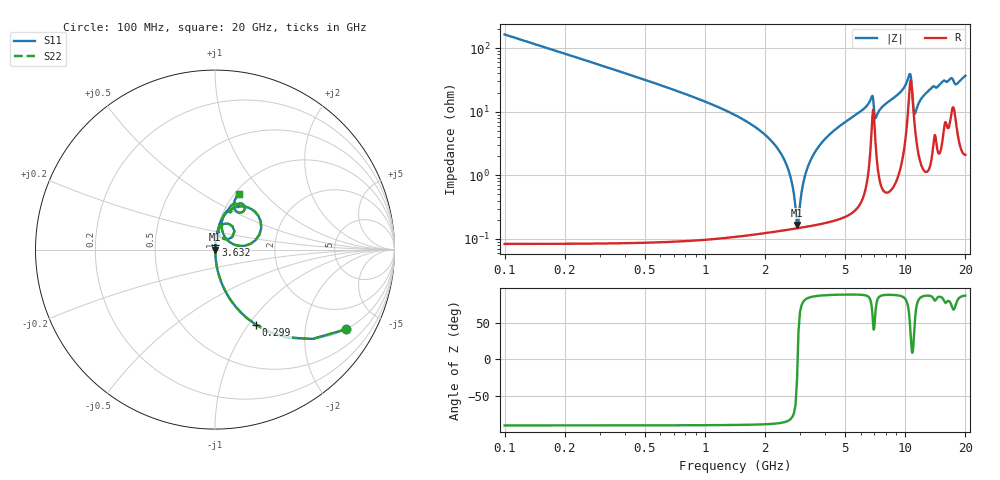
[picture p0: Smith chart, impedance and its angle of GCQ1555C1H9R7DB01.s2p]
!Murata Part Number: GCQ1555C1H9R7DB01
!These Parameters are Measured in Series Mode Connection
!Data Generated on Mar 13, 2026
!  o--ll--o
!Port1  Port2
!  o------o
!Operation Temp=25[degC], DC Bias Voltage=0[V]
!Freq. Start=100[MHz] Stop=20[GHz] 401[Steps]
# Hz S RI R 50
!Freq.(Hz) S11(Real) S11(Imag) S21(Real) S21(Imag) S12(Real) S12(Imag) S22(Real) S22(Imag)
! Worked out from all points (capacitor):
!   401 points, 100 MHz to 20 GHz, reference 50 ohm
!   read as one part in series: C = 9.7 pF near 199.5 MHz
!   lowest |Z| = 165 mohm at 2.886 GHz (marker M1)
!   series resonance near 2.905 GHz, so ESL is about 310 pH
!   S11 on the Smith chart (normalised r, x): 100 MHz: 1.00, -3.28; 299 MHz: 1.00, -1.09; 3.632 GHz: 1.00, +0.05; 20 GHz: 1.04, +0.74
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1e8  0.7286 -0.4444  0.2714 0.4444  0.2714 0.4444  0.7286 -0.4444
2.99e8  0.228 -0.4188  0.772 0.4188  0.772 0.4188  0.228 -0.4188
7.4675e8  0.0412 -0.1966  0.9588 0.1966  0.9588 0.1966  0.0412 -0.1966
2.33875e9  0.00194 -0.0248  0.9981 0.0248  0.9981 0.0248  0.00194 -0.0248
2.63725e9  0.00152 -0.011  0.9985 0.011  0.9985 0.011  0.00152 -0.011
2.886e9  0.00147 -0.000761  0.9985 0.000761  0.9985 0.000761  0.00147 -0.000761
2.9855e9  0.0015 0.0031  0.9985 -0.0031  0.9985 -0.0031  0.0015 0.0031
3.1845e9  0.00165 0.0105  0.9983 -0.0105  0.9983 -0.0105  0.00165 0.0105
3.43325e9  0.00198 0.0192  0.998 -0.0192  0.998 -0.0192  0.00198 0.0192
3.63225e9  0.00234 0.0259  0.9977 -0.0259  0.9977 -0.0259  0.00234 0.0259
4.478e9  0.00467 0.0521  0.9953 -0.0521  0.9953 -0.0521  0.00467 0.0521
6.7665e9  0.0582 0.1447  0.9418 -0.1447  0.9418 -0.1447  0.0582 0.1447
7.1645e9  0.029 0.0743  0.971 -0.0743  0.971 -0.0743  0.029 0.0743
1.005e10  0.0943 0.2282  0.9057 -0.2282  0.9057 -0.2282  0.0943 0.2282
1.059725e10  0.2547 0.1566  0.7453 -0.1566  0.7453 -0.1566  0.2547 0.1566
1.0846e10  0.1692 0.0221  0.8308 -0.0221  0.8308 -0.0221  0.1692 0.0221
1.11445e10  0.0647 0.0577  0.9353 -0.0577  0.9353 -0.0577  0.0647 0.0577
1.199025e10  0.0377 0.1483  0.9623 -0.1483  0.9623 -0.1483  0.0377 0.1483
1.338325e10  0.0617 0.2104  0.9383 -0.2104  0.9383 -0.2104  0.0617 0.2104
1.67165e10  0.1386 0.2575  0.8614 -0.2575  0.8614 -0.2575  0.1386 0.2575
1.79105e10  0.1186 0.2138  0.8814 -0.2138  0.8814 -0.2138  0.1186 0.2138
2e10  0.1332 0.3125  0.8668 -0.3125  0.8668 -0.3125  0.1332 0.3125
